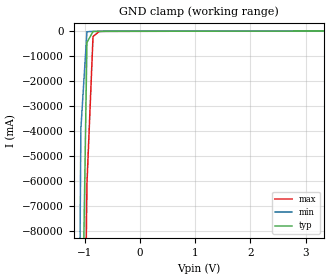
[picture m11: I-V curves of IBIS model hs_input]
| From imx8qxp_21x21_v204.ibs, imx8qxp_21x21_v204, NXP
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[Model]  hs_input
|   Model hs_input
| This model was characterised for following simulation conditions:
| Spice Models:
|  - Typ Condition
|   /project/usb2_ln28fdsoi/HS/s2ibis/HS_input/ln28fdsoi_lp2.combination ln28fdsoi_typ
|  - Min Condition
|   /project/usb2_ln28fdsoi/HS/s2ibis/HS_input/ln28fdsoi_lp2.combination ln28fdsoi_wcs
|  - Max Condition
|   /project/usb2_ln28fdsoi/HS/s2ibis/HS_input/ln28fdsoi_lp2.combination ln28fdsoi_bcs
Model_type Input
Vinl =   0.2100V
Vinh =   0.1900V
C_comp   2.8431pF   2.6338pF   3.0727pF
[Temperature Range]   27.0000   -40.0000   0.1050k
[Voltage Range]   3.3000V   3.0000V   3.6000V
[GND_clamp]
|Voltage   I(typ)   I(min)   I(max)
-3.6V     -10.68kA   -13.8kA    -8.465kA
-1.18V    -414.1A    -362.8A    -466.3A
-1.07V    -158.9A    -39.09A    -263.8A
-960mV    -4.47A     -193.6mA   -61.23A
-850mV    -89.47mA   -23.36mA   -2.124A
-740mV    -20.65mA   -18.81mA   -95.19mA
3.33V     76.47mA    76.35mA    76.04mA
